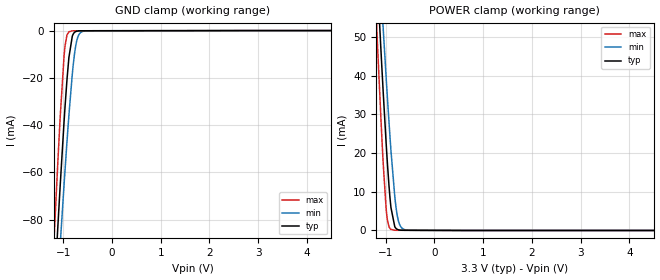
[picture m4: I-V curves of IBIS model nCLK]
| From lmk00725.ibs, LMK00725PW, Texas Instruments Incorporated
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|   Model nCLK
[Model]   nCLK
Model_type   Input
Vinl = 1.2
Vinh = 1.5
|   typ   min   max
|   (nom PVT)   (fast PVT)   (slow PVT)
C_comp   0.302p   0.289p   0.313p
[Voltage Range]   3.3   3.1   3.5
[Temperature Range]   45   125   -40
[Power Clamp Reference]   3.3   3.1   3.5
[GND Clamp Reference]   0   0   0
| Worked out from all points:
|   GND clamp passes 1 mA (typ) near -0.78 V on its own axis
|   POWER clamp passes 1 mA (typ) near -0.82 V on its own axis
[GND Clamp]
|   Voltage   I(typ)   I(min)   I(max)
-3.3V     -971.6mA   -905.8mA   -1.073A
-1.181V   -109.1mA   -130.1mA   -84.95mA
-1.112V   -83.21mA   -106.7mA   -55.88mA
-1.063V   -65.31mA   -90.39mA   -36.4mA
-973.5mV  -35.23mA   -61.95mA   -8.416mA
-924mV    -20.75mA   -47.02mA   -1.82mA
-884.4mV  -11.38mA   -35.77mA   -518.5uA
-815.1mV  -2.415mA   -18.52mA   -122.2uA
-745.8mV  -440.2uA   -6.626mA   -86.13uA
-676.5mV  -122.8uA   -1.646mA   -82.87uA
-577.5mV  -78.68uA   -233.6uA   -80.82uA
6.6V      0A         0A         0A
[POWER Clamp]
|   Voltage   I(typ)   I(min)   I(max)
-3.3V     640.7mA    598mA      708.5mA
-1.191V   69.22mA    82.71mA    54.03mA
-1.181V   66.75mA    80.48mA    51.22mA
-1.092V   44.99mA    60.72mA    27.01mA
-1.053V   35.75mA    52.17mA    17.31mA
-973.5mV  18.74mA    35.74mA    3.364mA
-894.3mV  5.963mA    20.77mA    276.9uA
-815.1mV  970.5uA    8.779mA    59.59uA
-765.6mV  308.6uA    3.979mA    51.59uA
-706.2mV  93.69uA    1.281mA    48.72uA
-607.2mV  49.5uA     200.9uA    44.84uA
6.6V      0A         0A         0A
